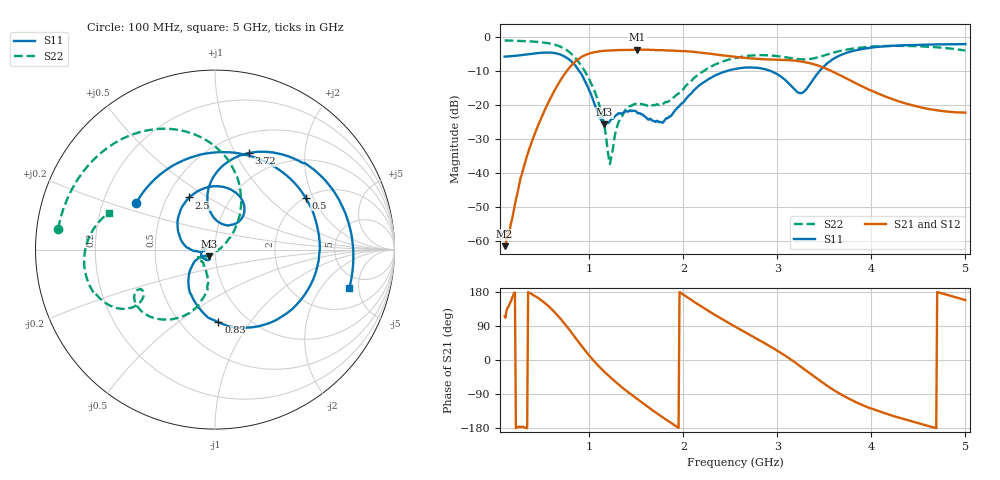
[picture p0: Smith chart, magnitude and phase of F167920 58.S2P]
!  2-Port S-parameters saved by WinCal
! VAR MeasName=S-Parameters (CALIBRATED_DATA) read from VNA (N5242A)
! VAR MeasDate=2016-11-22 9:58:24
! VAR NAME=F167920 58
! VAR FILENAME=F167920 58.S2P
! VAR DATE=2016-11-22 9:58:24
! VAR PHYS_PORTS=1,2
# Hz S DB R 50
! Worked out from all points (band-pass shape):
!   491 points, 100 MHz to 5 GHz, reference 50 ohm
!   highest |S21| = -3.80 dB at 1.51 GHz (marker M1); lowest = -61.7 dB at 100 MHz (marker M2)
!   |S21| within 3 dB of the highest: 874.4 MHz to 3.033 GHz (2.159 GHz wide, 110 % of centre)
!   lowest |S11| = -25.8 dB at 1.16 GHz (marker M3), VSWR 1.11, Z = 46.5 - j3.46 ohm
!   |S11| at or under -10 dB: 891 MHz to 2.474 GHz (1.583 GHz wide, 94.1 % of centre); 2.92 GHz to 3.452 GHz (532 MHz wide, 16.7 % of centre)
!   |S22| runs from -37.5 to -1.1 dB; largest |S21 - S12| = 0.0016
!   S11 on the Smith chart (normalised r, x): 100 MHz: 0.35, +0.24; 500 MHz: 2.01, +1.76; 830 MHz: 0.74, -0.72; 2.5 GHz: 0.64, +0.42; 3.72 GHz: 0.71, +1.13; 5 GHz: 3.66, -3.92
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1e8  -5.86 149.5  -61.66 115.8  -61.63 112.7  -1.10 172.4
3.1e8  -5.29 87.2  -37.76 -177.9  -37.66 -177.2  -1.28 155.7
5e8  -4.70 29.9  -23.26 155.9  -23.26 155.9  -1.66 137.0
6.5e8  -4.92 -20.1  -14.87 121.3  -14.86 121.4  -2.48 116.8
7.4e8  -5.85 -53.1  -10.90 95.3  -10.90 95.4  -3.60 101.5
8.3e8  -7.84 -87.3  -7.91 66.3  -7.89 66.4  -5.57 84.3
9.2e8  -11.13 -120.3  -5.90 36.8  -5.89 36.8  -8.75 67.4
1.06e9  -20.09 -152.6  -4.53 -5.4  -4.53 -5.4  -16.25 45.3
1.16e9  -25.79 -133.6  -4.15 -31.0  -4.15 -31.1  -26.10 25.5
1.22e9  -24.87 -120.1  -4.04 -44.9  -4.04 -44.9  -37.49 -52.5
1.33e9  -22.66 -132.7  -3.90 -68.4  -3.90 -68.4  -24.26 -141.1
1.51e9  -22.32 -170.6  -3.80 -103.0  -3.80 -103.0  -19.96 -155.8
1.74e9  -25.19 175.8  -3.93 -144.0  -3.93 -144.1  -20.11 -137.9
2.06e9  -17.30 179.6  -4.36 162.6  -4.35 162.6  -13.60 -101.8
2.5e9  -9.79 116.3  -5.77 95.3  -5.79 95.2  -6.61 -123.6
2.55e9  -9.50 109.2  -5.92 88.3  -5.94 88.3  -6.28 -126.6
3.04e9  -11.76 51.2  -6.80 18.4  -6.82 18.5  -5.84 -151.4
3.24e9  -16.60 69.0  -7.24 -16.0  -7.24 -15.9  -6.63 -151.6
3.37e9  -13.03 97.9  -7.95 -39.7  -7.96 -39.6  -6.46 -147.0
3.72e9  -4.89 70.8  -12.06 -96.8  -12.10 -96.6  -3.87 -149.7
4.19e9  -2.72 29.6  -18.04 -144.3  -18.07 -143.9  -2.70 -168.0
5e9  -2.18 -15.8  -22.34 157.9  -22.32 158.4  -4.09 160.9
